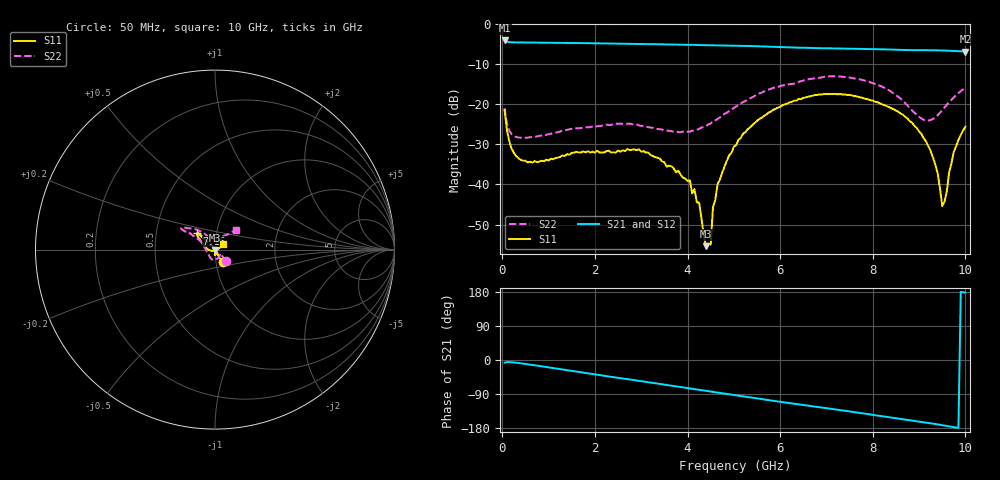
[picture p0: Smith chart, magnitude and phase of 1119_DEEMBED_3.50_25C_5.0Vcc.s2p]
!Hittite Microwave Corp.
!Digital Attenuator/PhaseShifter Rev 1.4.0
!Filename: C:\DATA\DATA\1119_DEEMBED_3.50_25C_5.0Vcc.s2p
!VNA ID: Agilent Technologies,N5224A,MY51441122,A.10.45.03
!Device type:
!2 Port Calibration.
!Temp(C): 25
!Lot Number:
!Serial Number:
!Operator:
!Misc:
!Attenuator:  3.500
# GHZ S DB R 50.0
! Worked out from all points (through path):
!   200 points, 50 MHz to 10 GHz, reference 50 ohm
!   highest |S21| = -4.07 dB at 50 MHz (marker M1); lowest = -6.8 dB at 10 GHz (marker M2)
!   group delay of S21, straight-line fit = 49.6 ps
!   lowest |S11| = -55.4 dB at 4.4 GHz (marker M3), VSWR 1.00, Z = 50 - j0.168 ohm
!   |S11| at or under -10 dB: start of sweep to end of sweep
!   |S22| runs from -28.4 to -13.0 dB; largest |S21 - S12| = 0.0015
!   S11 on the Smith chart (normalised r, x): 50 MHz: 1.08, -0.16; 7.15 GHz: 0.81, +0.15; 10 GHz: 1.09, +0.07
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0.05  -21.44 -57.7  -4.07 -7.0  -4.07 -7.0  -21.00 -45.1
0.2  -31.02 -57.4  -4.52 -5.8  -4.52 -5.9  -27.44 -35.5
0.4  -33.85 -51.5  -4.57 -8.7  -4.57 -8.7  -28.34 -32.4
1.75  -31.74 -89.4  -4.73 -33.2  -4.74 -33.3  -25.78 -73.5
2.95  -31.23 -88.8  -4.96 -54.9  -4.97 -55.0  -25.27 -113.8
3.4  -33.53 -86.2  -5.01 -63.2  -5.02 -63.2  -26.22 -128.7
4.15  -41.15 -59.8  -5.19 -76.9  -5.20 -76.9  -26.51 -168.4
4.25  -44.56 -54.4  -5.22 -78.6  -5.23 -78.7  -26.15 -174.6
4.4  -55.39 -81.7  -5.25 -81.3  -5.26 -81.4  -25.46 175.2
4.5  -55.00 129.6  -5.28 -83.0  -5.30 -83.1  -24.79 169.2
4.55  -45.65 127.3  -5.28 -84.0  -5.30 -84.0  -24.20 166.0
4.65  -39.84 124.1  -5.30 -85.8  -5.32 -85.8  -23.66 161.2
5.05  -30.19 130.2  -5.38 -93.0  -5.40 -93.0  -20.55 149.7
5.75  -22.07 135.6  -5.61 -105.8  -5.63 -105.9  -16.33 147.4
6.7  -17.85 135.7  -5.94 -121.9  -5.95 -121.9  -13.58 148.4
7.15  -17.44 137.8  -6.05 -129.5  -6.06 -129.6  -13.00 146.9
8.35  -20.69 148.8  -6.32 -150.9  -6.32 -150.9  -16.50 132.0
9.15  -29.20 -175.8  -6.50 -165.0  -6.51 -165.1  -24.07 101.2
9.400001  -37.14 -149.9  -6.53 -169.9  -6.55 -170.0  -22.75 70.6
9.5  -45.38 -110.5  -6.57 -172.0  -6.58 -172.0  -21.47 60.7
9.75  -31.84 20.9  -6.69 -177.1  -6.70 -177.1  -18.27 47.7
10  -25.55 36.9  -6.84 177.8  -6.85 177.8  -15.94 44.0
